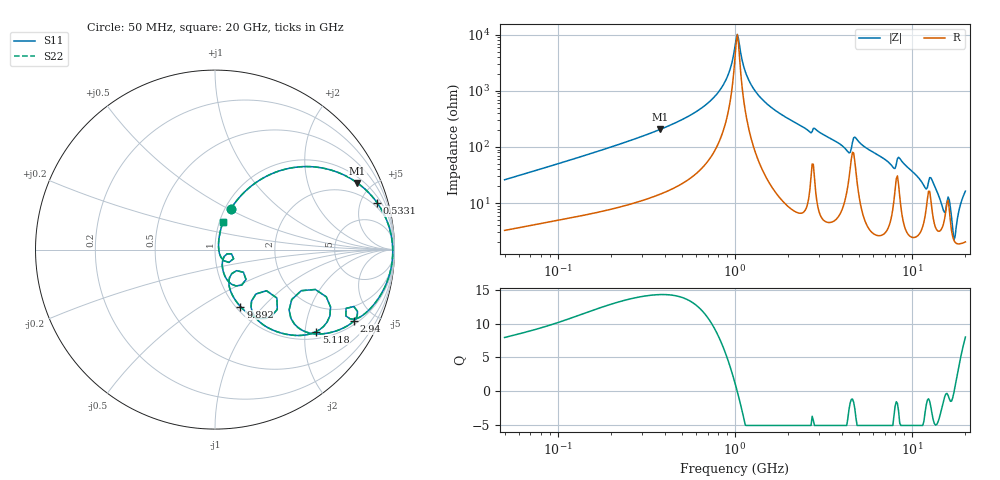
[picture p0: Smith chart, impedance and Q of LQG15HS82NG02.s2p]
!Murata Part Number: LQG15HS82NG02
!These Parameters are Measured in Series Mode Connection
!  o--[Z]--o
!Port1  Port2
!  o-------o
!Freq. Start=50[MHz] Stop=20[GHz], 401[Steps]
# Hz S RI R 50
!Freq.(Hz) S11(Real) S11(Imag) S21(Real) S21(Imag) S12(Real) S12(Imag) S22(Real) S22(Imag)
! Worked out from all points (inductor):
!   401 points, 50 MHz to 20 GHz, reference 50 ohm
!   read as one part in series: L = 80.8 nH near 51.52 MHz
!   highest Q = 14.3 at 377.7 MHz (marker M1), where L = 86.4 nH
!   self-resonance near 1.015 GHz
!   S11 on the Smith chart (normalised r, x): 50 MHz: 1.07, +0.52; 533.1 MHz: 1.50, +6.77; 2.94 GHz: 1.17, -3.81; 5.118 GHz: 1.19, -2.29; 9.892 GHz: 1.05, -0.76; 20 GHz: 1.04, +0.32
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5e7  0.0885 0.228  0.9115 -0.228  0.9115 -0.228  0.0885 0.228
1.364002e8  0.3301 0.4283  0.6699 -0.4283  0.6699 -0.4283  0.3301 0.4283
3.721004e8  0.7868 0.376  0.2132 -0.376  0.2132 -0.376  0.7868 0.376
3.777159e8  0.7927 0.3718  0.2073 -0.3718  0.2073 -0.3718  0.7927 0.3718
5.330693e8  0.9039 0.2601  0.0961 -0.2601  0.0961 -0.2601  0.9039 0.2601
8.230629e8  0.979 0.0921  0.021 -0.0921  0.021 -0.0921  0.979 0.0921
1e9  0.9898 0.0123  0.0102 -0.0123  0.0102 -0.0123  0.9898 0.0123
1.045961e9  0.9903 -0.00633  0.00966 0.00633  0.00966 0.00633  0.9903 -0.00633
1.179116e9  0.9881 -0.0564  0.0119 0.0564  0.0119 0.0564  0.9881 -0.0564
1.411297e9  0.9741 -0.1324  0.0259 0.1324  0.0259 0.1324  0.9741 -0.1324
2.728004e9  0.7298 -0.3277  0.2702 0.3277  0.2702 0.3277  0.7298 -0.3277
2.940159e9  0.7747 -0.3964  0.2253 0.3964  0.2253 0.3964  0.7747 -0.3964
4.34015e9  0.4227 -0.3824  0.5773 0.3824  0.5773 0.3824  0.4227 -0.3824
5.117541e9  0.5645 -0.4567  0.4355 0.4567  0.4355 0.4567  0.5645 -0.4567
7.442007e9  0.2287 -0.3824  0.7713 0.3824  0.7713 0.3824  0.2287 -0.3824
9.892087e9  0.1418 -0.3177  0.8582 0.3177  0.8582 0.3177  0.1418 -0.3177
1.183995e10  0.0812 -0.1553  0.9188 0.1553  0.9188 0.1553  0.0812 -0.1553
1.295331e10  0.1173 -0.2025  0.8827 0.2025  0.8827 0.2025  0.1173 -0.2025
1.504638e10  0.0441 -0.0547  0.9559 0.0547  0.9559 0.0547  0.0441 -0.0547
1.621653e10  0.0779 -0.0713  0.9221 0.0713  0.9221 0.0713  0.0779 -0.0713
1.721783e10  0.0213 -0.00359  0.9787 0.00359  0.9787 0.00359  0.0213 -0.00359
2e10  0.0441 0.1521  0.9559 -0.1521  0.9559 -0.1521  0.0441 0.1521
